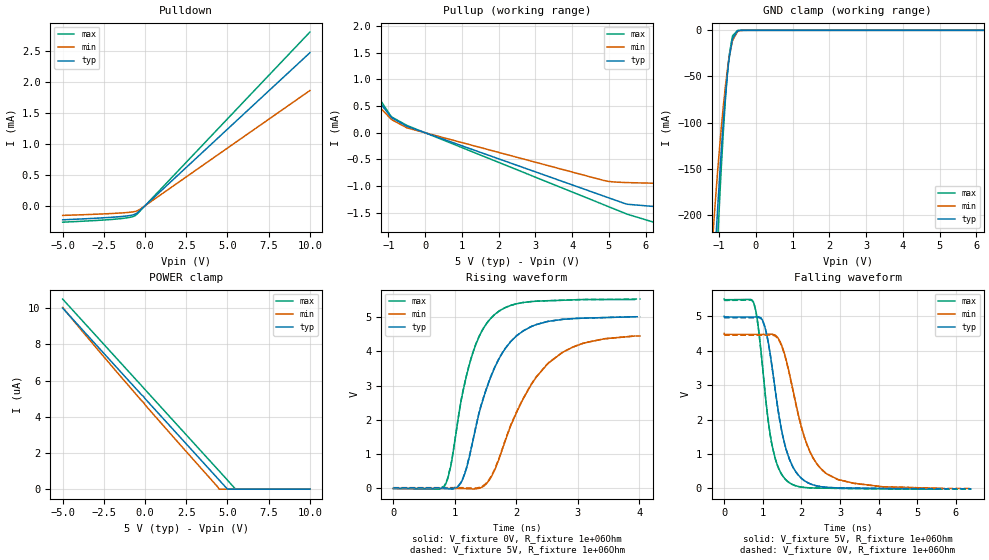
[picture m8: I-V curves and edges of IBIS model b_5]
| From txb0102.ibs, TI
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|   b_5 Model
[Model]   b_5
Model_type   I/O
Polarity   Non-Inverting
Enable   Active-High
Vinl = 1.75
Vinh = 3.25
Vmeas = 2.5
Vref = 0
Cref = 2pF
Rref = 1e6
|   typ   min   max
|   (nom PVT)   (fast PVT)   (slow PVT)
C_comp   1.016e-11   1.016e-11   1.022e-11
[Model spec]
|subparameter
Vinl   1.75   1.575   1.925
Vinh   3.25   2.925   3.575
| Where nom  PVT is Nominal Process, 5V, 27C
|   Fast PVT is Strong Process,  5.5V, -40C
|   Slow PVT is Weak Process,   4.5V, 125C
[Voltage Range]   5   4.5   5.5
|Junction Temperature
[Temperature Range]   27   125   -40
[Pullup Reference]   5   4.5   5.5
[Pulldown Reference]   0   0   0
[Power Clamp Reference]   5   4.5   5.5
[GND Clamp Reference]   0   0   0
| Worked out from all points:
|   slope of the pulldown table from 0 to 0.75 V, typ, clamps not added: 4.05 kohm
|   slope of the pullup table from 0 to 0.75 V, typ, clamps not added: 4.09 kohm
|   GND clamp passes 1 mA (typ) near -0.51 V on its own axis
|   falling waveform, V_fixture 5V, R_fixture 1e+06Ohm: 20-80 % time 468ps typ, 662ps min, 362ps max; typ from 5 V to -0.009 V
|   rising waveform, V_fixture 0V, R_fixture 1e+06Ohm: 20-80 % time 546ps typ, 747ps min, 413ps max; typ from 0 V to 5.01 V
|   rising waveform, V_fixture 5V, R_fixture 1e+06Ohm: 20-80 % time 545ps typ, 746ps min, 415ps max; typ from 0.02 V to 5.01 V
|   falling waveform, V_fixture 0V, R_fixture 1e+06Ohm: 20-80 % time 467ps typ, 659ps min, 361ps max; typ from 4.96 V to -0.009 V
[Pulldown]
|   Voltage   I(typ)   I(min)   I(max)
-5V       -227.6uA   -156.7uA   -266uA
-1.652V   -179.5uA   -120.6uA   -213.4uA
-919mV    -158.2uA   -105.6uA   -187.7uA
-560mV    -130.2uA   -90.19uA   -153.1uA
-234.5mV  -57.89uA   -43.53uA   -65.7uA
10V       2.466mA    1.857mA    2.799mA
[GND Clamp]
|   Voltage   I(typ)   I(min)   I(max)
-5V       -4.689A    -3.794A    -5.371A
-1.2V     -311mA     -240.4mA   -375.4mA
-1.112V   -243.9mA   -190.4mA   -291.8mA
-1.101V   -235.5mA   -184.2mA   -281.3mA
-1.031V   -187mA     -148.1mA   -220.5mA
-955mV    -138.6mA   -111.9mA   -159.6mA
-885mV    -98.75mA   -81.96mA   -109.8mA
-831mV    -71.66mA   -61.37mA   -76.3mA
-748.5mV  -37.66mA   -34.99mA   -35.71mA
-644mV    -10.75mA   -12.52mA   -7.368mA
-500mV    -653.7uA   -1.408mA   -181.8uA
10V       0A         0A         0A
[Pullup]
|   Voltage   I(typ)   I(min)   I(max)
-5V       9.23mA     5.565mA    13.12mA
-2.24V    2.613mA    2.382mA    2.793mA
-2.026V   1.873mA    1.812mA    2.14mA
-1.893V   1.548mA    1.482mA    1.825mA
-1.728V   1.24mA     1.125mA    1.475mA
-1.359V   713.4uA    601.3uA    816.5uA
-941mV    306.2uA    266.3uA    322.7uA
-459.5mV  112.4uA    85.46uA    127.7uA
4.895V    -1.197mA   -900.7uA   -1.361mA
5.503V    -1.343mA   -935.8uA   -1.53mA
6.374V    -1.393mA   -950.4uA   -1.712mA
10V       -1.438mA   -981.1uA   -1.778mA
[POWER Clamp]
|   Voltage   I(typ)   I(min)   I(max)
-5V       10uA       10.04uA    10.5uA
-1.738V   6.739uA    6.497uA    7.238uA
4.495V    505.1nA    0A         1.005uA
4.995V    0A         0A         505nA
5.49V     0A         0A         0A
10V       0A         0A         0A
[Ramp]
R_load = 1e+06
|   typ   min   max
dV/dt_r   2.98515/5.36681e-10   2.68086/7.51427e-10   3.28565/4.06654e-10
dV/dt_f   2.98433/4.61109e-10   2.68317/6.58288e-10   3.28333/3.53297e-10
[Falling Waveform]
V_fixture = 5V
V_fixture_min = 4.5V
V_fixture_max = 5.5V
R_fixture = 1e+06Ohm
|   Time   V(typ)   V(min)   V(max)
0s        5V         4.5V       5.5V
760ps     4.978V     4.475V     5.409V
864ps     4.984V     4.475V     4.856V
1.032ns   4.782V     4.474V     3.099V
1.224ns   3.667V     4.48V      1.356V
1.444ns   1.958V     4.273V     505mV
1.604ns   1.141V     3.742V     245.7mV
2.092ns   216.8mV    1.446V     28.65mV
2.634ns   35.29mV    444.5mV    7.68mV
5.634ns   -9.003mV   2.374mV    -19.54mV
[Rising Waveform]
V_fixture = 0V
V_fixture_min = 0V
V_fixture_max = 0V
R_fixture = 1e+06Ohm
|   Time   V(typ)   V(min)   V(max)
0s        136.2nV    26.93uV    78.3nV
828ps     -1.51mV    -46.4uV    60.65mV
932ps     -15.67mV   164.3uV    646.1mV
1.052ns   53.57mV    616uV      2.017V
1.236ns   923.3mV    -10.06mV   3.618V
1.414ns   2.335V     17.82mV    4.503V
1.656ns   3.56V      575.6mV    5.086V
2.102ns   4.585V     2.587V     5.42V
2.526ns   4.875V     3.664V     5.476V
3.92ns    5.007V     4.445V     5.511V
[Rising Waveform]
V_fixture = 5V
V_fixture_min = 4.5V
V_fixture_max = 5.5V
R_fixture = 1e+06Ohm
|   Time   V(typ)   V(min)   V(max)
0s        20.09mV    23.89mV    19.49mV
826ps     18.75mV    23.81mV    74.89mV
932ps     4.531mV    24.02mV    666.1mV
1.056ns   80.96mV    24.44mV    2.083V
1.236ns   943.5mV    13.86mV    3.632V
1.416ns   2.365V     43.08mV    4.518V
1.656ns   3.571V     599.9mV    5.09V
2.1ns     4.586V     2.594V     5.421V
2.524ns   4.876V     3.668V     5.476V
4.02ns    5.008V     4.445V     5.523V
[Falling Waveform]
V_fixture = 0V
V_fixture_min = 0V
V_fixture_max = 0V
R_fixture = 1e+06Ohm
|   Time   V(typ)   V(min)   V(max)
0s        4.959V     4.451V     5.461V
762ps     4.958V     4.451V     5.384V
894ps     4.965V     4.451V     4.581V
1.032ns   4.761V     4.45V      3.082V
1.244ns   3.488V     4.456V     1.23V
1.478ns   1.737V     4.164V     430.7mV
1.676ns   886.8mV    3.386V     174.8mV
2.138ns   182.8mV    1.287V     23.9mV
2.654ns   32.68mV    422.9mV    7.34mV
6.4ns     -9.153mV   2.135mV    -20.11mV
